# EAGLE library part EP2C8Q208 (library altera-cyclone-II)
EP2C8Q208 Auto generated by make-symbol-device-package-bsdl.ulp Rev. 19 Tip: Use split-device-symbol.ulp to generate a Device with multiple small symbols! Read HELP. Source: EP2C8Q208.BSD
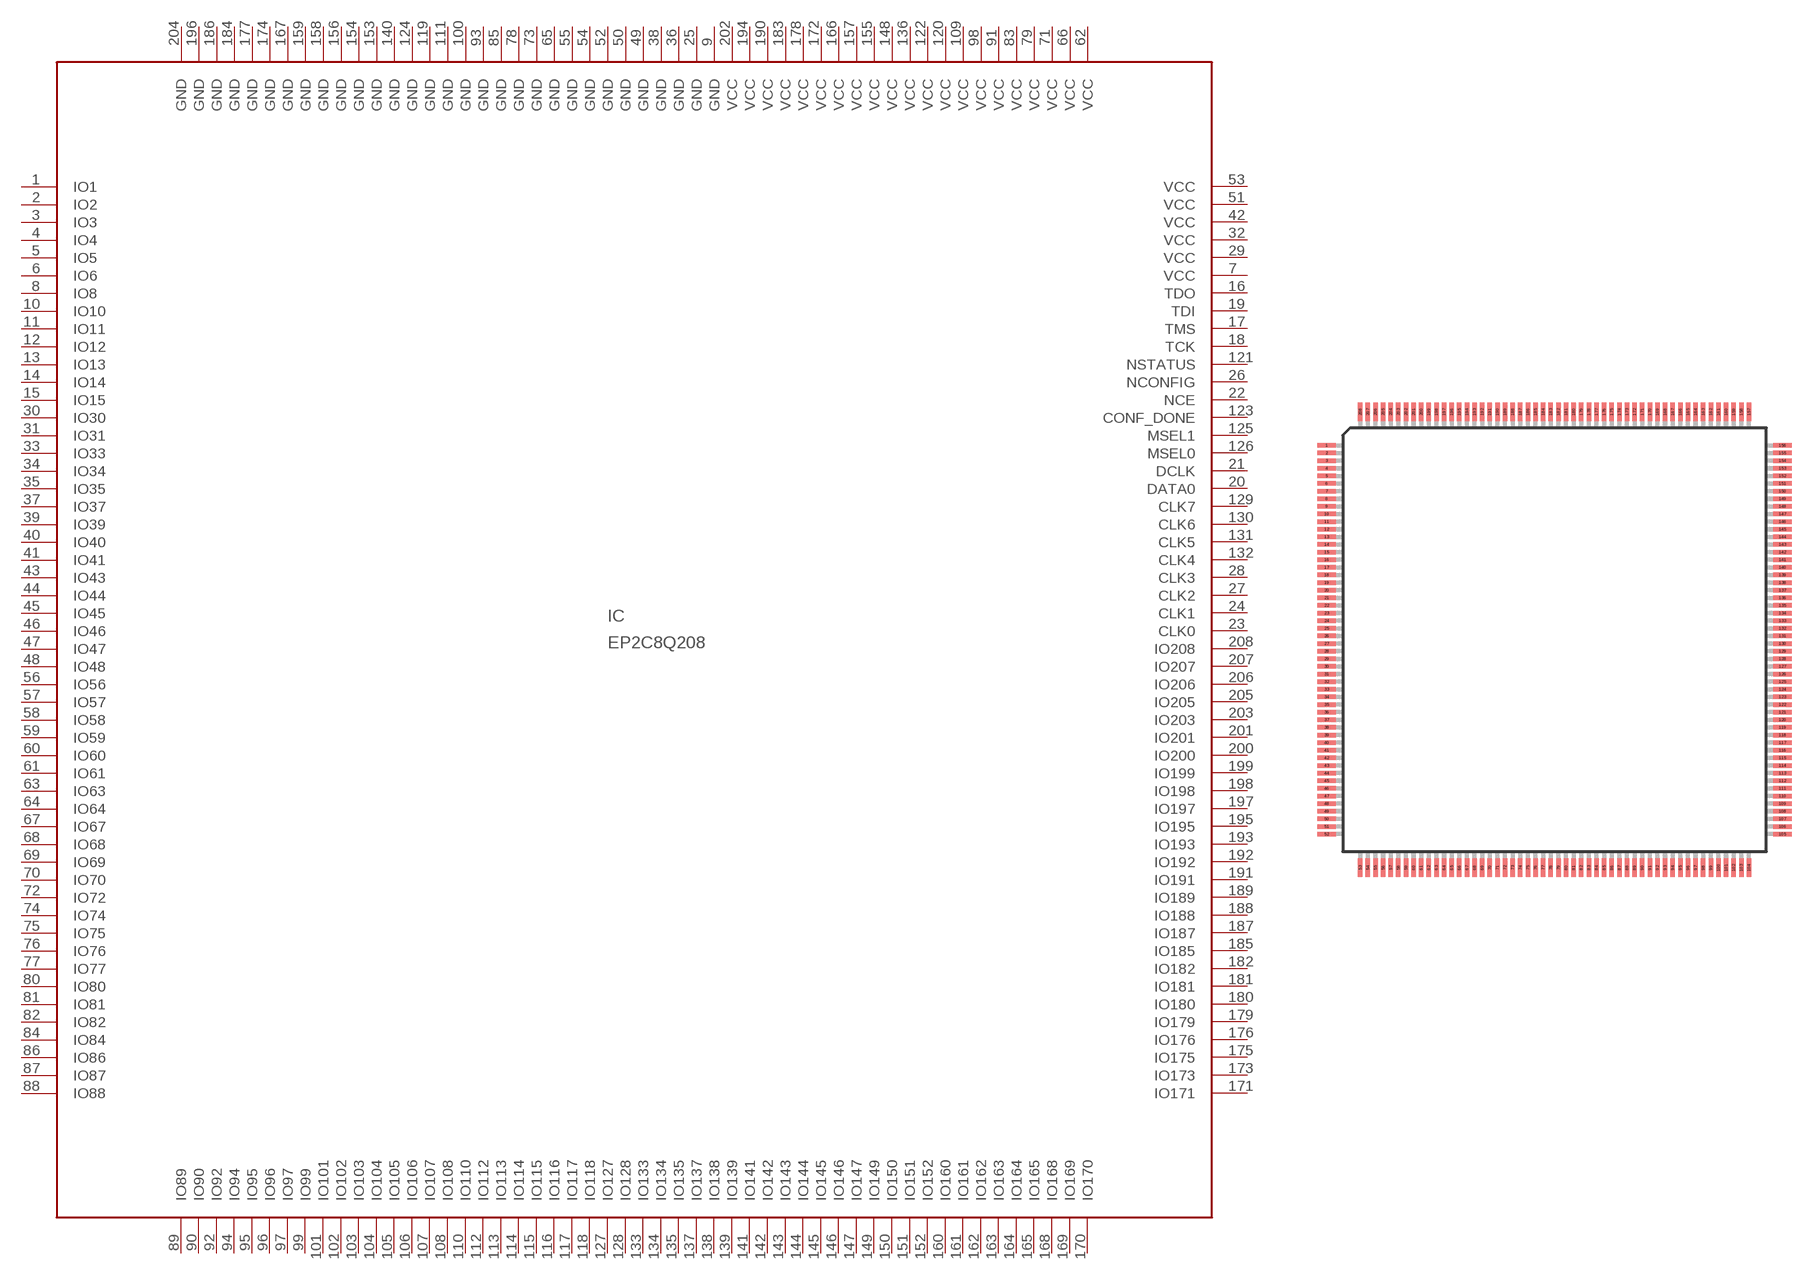
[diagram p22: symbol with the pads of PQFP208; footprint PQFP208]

Designator prefix IC

## EP2C8Q208 (MPN: EP2C8Q208C8N; OC_FARNELL: 1663194; OC_NEWARK: 51R0575)  [PQFP208]
1  IO1  out
2  IO2  out
3  IO3
4  IO4
5  IO5
6  IO6
7  VCC  pwr
8  IO8
9  GND  pwr
10  IO10
11  IO11
12  IO12
13  IO13
14  IO14
15  IO15
16  TDO  out
17  TMS  in
18  TCK  in
19  TDI  in
20  DATA0
21  DCLK
22  NCE  in
23  CLK0
24  CLK1
25  GND  pwr
26  NCONFIG  in
27  CLK2
28  CLK3
29  VCC  pwr
30  IO30
31  IO31
32  VCC  pwr
33  IO33
34  IO34
35  IO35
36  GND  pwr
37  IO37
38  GND  pwr
39  IO39
40  IO40
41  IO41
42  VCC  pwr
43  IO43
44  IO44
45  IO45
46  IO46
47  IO47
48  IO48
49  GND  pwr
50  GND  pwr
51  VCC  pwr
52  GND  pwr
53  VCC  pwr
54  GND  pwr
55  GND  pwr
56  IO56
57  IO57
58  IO58
59  IO59
60  IO60
61  IO61
62  VCC  pwr
63  IO63
64  IO64
65  GND  pwr
66  VCC  pwr
67  IO67
68  IO68
69  IO69
70  IO70
71  VCC  pwr
72  IO72
73  GND  pwr
74  IO74
75  IO75
76  IO76
77  IO77
78  GND  pwr
79  VCC  pwr
80  IO80
81  IO81
82  IO82
83  VCC  pwr
84  IO84
85  GND  pwr
86  IO86
87  IO87
88  IO88
89  IO89
90  IO90
91  VCC  pwr
92  IO92
93  GND  pwr
94  IO94
95  IO95
96  IO96
97  IO97
98  VCC  pwr
99  IO99
100  GND  pwr
101  IO101
102  IO102
103  IO103
104  IO104
105  IO105
106  IO106
107  IO107
108  IO108
109  VCC  pwr
110  IO110
111  GND  pwr
112  IO112
113  IO113
114  IO114
115  IO115
116  IO116
117  IO117
118  IO118
119  GND  pwr
120  VCC  pwr
121  NSTATUS  in
122  VCC  pwr
123  CONF_DONE  in
124  GND  pwr
125  MSEL1  in
126  MSEL0  in
127  IO127
128  IO128
129  CLK7
130  CLK6
131  CLK5
132  CLK4
133  IO133
134  IO134
135  IO135
136  VCC  pwr
137  IO137
138  IO138
139  IO139
140  GND  pwr
141  IO141
142  IO142
143  IO143
144  IO144
145  IO145
146  IO146
147  IO147
148  VCC  pwr
149  IO149
150  IO150
151  IO151
152  IO152
153  GND  pwr
154  GND  pwr
155  VCC  pwr
156  GND  pwr
157  VCC  pwr
158  GND  pwr
159  GND  pwr
160  IO160
161  IO161
162  IO162
163  IO163
164  IO164
165  IO165
166  VCC  pwr
167  GND  pwr
168  IO168
169  IO169
170  IO170
171  IO171
172  VCC  pwr
173  IO173
174  GND  pwr
175  IO175
176  IO176
177  GND  pwr
178  VCC  pwr
179  IO179
180  IO180
181  IO181
182  IO182
183  VCC  pwr
184  GND  pwr
185  IO185
186  GND  pwr
187  IO187
188  IO188
189  IO189
190  VCC  pwr
191  IO191
192  IO192
193  IO193
194  VCC  pwr
195  IO195
196  GND  pwr
197  IO197
198  IO198
199  IO199
200  IO200
201  IO201
202  VCC  pwr
203  IO203
204  GND  pwr
205  IO205
206  IO206
207  IO207
208  IO208

## Footprint PQFP208 (pad centres in mm)
PQFP208 Auto generated by make-symbol-device-package-bsdl.ulp Rev. 19 Source: www.altera.com .. cyc2_cii51015.pdf
smd 1.2 x 0.3: 1 -14.95,12.75; 2 -14.95,12.25; 3 -14.95,11.75; 4 -14.95,11.25; 5 -14.95,10.75; 6 -14.95,10.25; 7 -14.95,9.75; 8 -14.95,9.25; 9 -14.95,8.75; 10 -14.95,8.25; 11 -14.95,7.75; 12 -14.95,7.25; 13 -14.95,6.75; 14 -14.95,6.25; 15 -14.95,5.75; 16 -14.95,5.25; 17 -14.95,4.75; 18 -14.95,4.25; 19 -14.95,3.75; 20 -14.95,3.25; 21 -14.95,2.75; 22 -14.95,2.25; 23 -14.95,1.75; 24 -14.95,1.25; 25 -14.95,0.75; 26 -14.95,0.25; 27 -14.95,-0.25; 28 -14.95,-0.75; 29 -14.95,-1.25; 30 -14.95,-1.75; 31 -14.95,-2.25; 32 -14.95,-2.75; 33 -14.95,-3.25; 34 -14.95,-3.75; 35 -14.95,-4.25; 36 -14.95,-4.75; 37 -14.95,-5.25; 38 -14.95,-5.75; 39 -14.95,-6.25; 40 -14.95,-6.75; 41 -14.95,-7.25; 42 -14.95,-7.75; 43 -14.95,-8.25; 44 -14.95,-8.75; 45 -14.95,-9.25; 46 -14.95,-9.75; 47 -14.95,-10.25; 48 -14.95,-10.75; 49 -14.95,-11.25; 50 -14.95,-11.75; 51 -14.95,-12.25; 52 -14.95,-12.75; 105 14.95,-12.75; 106 14.95,-12.25; 107 14.95,-11.75; 108 14.95,-11.25; 109 14.95,-10.75; 110 14.95,-10.25; 111 14.95,-9.75; 112 14.95,-9.25; 113 14.95,-8.75; 114 14.95,-8.25; 115 14.95,-7.75; 116 14.95,-7.25; 117 14.95,-6.75; 118 14.95,-6.25; 119 14.95,-5.75; 120 14.95,-5.25; 121 14.95,-4.75; 122 14.95,-4.25; 123 14.95,-3.75; 124 14.95,-3.25; 125 14.95,-2.75; 126 14.95,-2.25; 127 14.95,-1.75; 128 14.95,-1.25; 129 14.95,-0.75; 130 14.95,-0.25; 131 14.95,0.25; 132 14.95,0.75; 133 14.95,1.25; 134 14.95,1.75; 135 14.95,2.25; 136 14.95,2.75; 137 14.95,3.25; 138 14.95,3.75; 139 14.95,4.25; 140 14.95,4.75; 141 14.95,5.25; 142 14.95,5.75; 143 14.95,6.25; 144 14.95,6.75; 145 14.95,7.25; 146 14.95,7.75; 147 14.95,8.25; 148 14.95,8.75; 149 14.95,9.25; 150 14.95,9.75; 151 14.95,10.25; 152 14.95,10.75; 153 14.95,11.25; 154 14.95,11.75; 155 14.95,12.25; 156 14.95,12.75
smd 0.3 x 1.2: 53 -12.75,-14.95; 54 -12.25,-14.95; 55 -11.75,-14.95; 56 -11.25,-14.95; 57 -10.75,-14.95; 58 -10.25,-14.95; 59 -9.75,-14.95; 60 -9.25,-14.95; 61 -8.75,-14.95; 62 -8.25,-14.95; 63 -7.75,-14.95; 64 -7.25,-14.95; 65 -6.75,-14.95; 66 -6.25,-14.95; 67 -5.75,-14.95; 68 -5.25,-14.95; 69 -4.75,-14.95; 70 -4.25,-14.95; 71 -3.75,-14.95; 72 -3.25,-14.95; 73 -2.75,-14.95; 74 -2.25,-14.95; 75 -1.75,-14.95; 76 -1.25,-14.95; 77 -0.75,-14.95; 78 -0.25,-14.95; 79 0.25,-14.95; 80 0.75,-14.95; 81 1.25,-14.95; 82 1.75,-14.95; 83 2.25,-14.95; 84 2.75,-14.95; 85 3.25,-14.95; 86 3.75,-14.95; 87 4.25,-14.95; 88 4.75,-14.95; 89 5.25,-14.95; 90 5.75,-14.95; 91 6.25,-14.95; 92 6.75,-14.95; 93 7.25,-14.95; 94 7.75,-14.95; 95 8.25,-14.95; 96 8.75,-14.95; 97 9.25,-14.95; 98 9.75,-14.95; 99 10.25,-14.95; 100 10.75,-14.95; 101 11.25,-14.95; 102 11.75,-14.95; 103 12.25,-14.95; 104 12.75,-14.95; 157 12.75,14.95; 158 12.25,14.95; 159 11.75,14.95; 160 11.25,14.95; 161 10.75,14.95; 162 10.25,14.95; 163 9.75,14.95; 164 9.25,14.95; 165 8.75,14.95; 166 8.25,14.95; 167 7.75,14.95; 168 7.25,14.95; 169 6.75,14.95; 170 6.25,14.95; 171 5.75,14.95; 172 5.25,14.95; 173 4.75,14.95; 174 4.25,14.95; 175 3.75,14.95; 176 3.25,14.95; 177 2.75,14.95; 178 2.25,14.95; 179 1.75,14.95; 180 1.25,14.95; 181 0.75,14.95; 182 0.25,14.95; 183 -0.25,14.95; 184 -0.75,14.95; 185 -1.25,14.95; 186 -1.75,14.95; 187 -2.25,14.95; 188 -2.75,14.95; 189 -3.25,14.95; 190 -3.75,14.95; 191 -4.25,14.95; 192 -4.75,14.95; 193 -5.25,14.95; 194 -5.75,14.95; 195 -6.25,14.95; 196 -6.75,14.95; 197 -7.25,14.95; 198 -7.75,14.95; 199 -8.25,14.95; 200 -8.75,14.95; 201 -9.25,14.95; 202 -9.75,14.95; 203 -10.25,14.95; 204 -10.75,14.95; 205 -11.25,14.95; 206 -11.75,14.95; 207 -12.25,14.95; 208 -12.75,14.95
